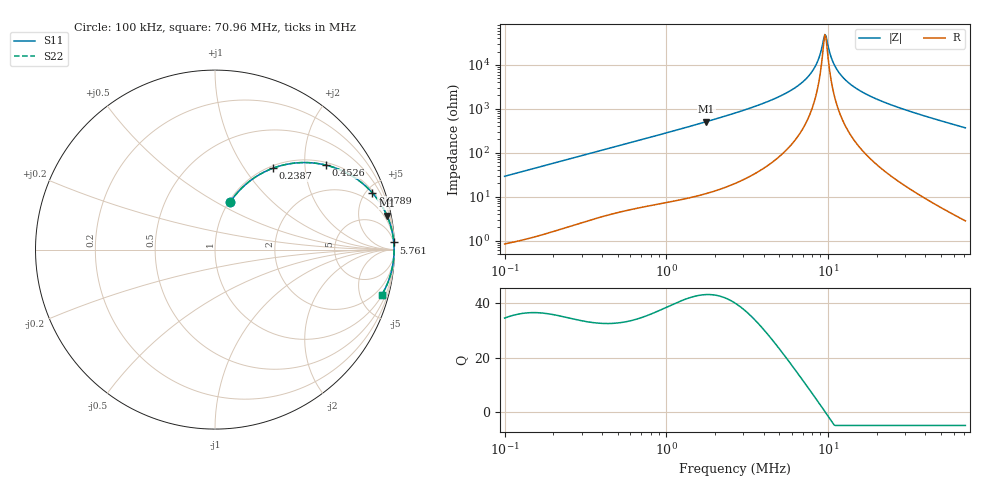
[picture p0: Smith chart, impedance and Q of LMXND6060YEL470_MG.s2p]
! LMXND6060YEL470_MG  S-PARAMETER MODEL  ( General Type )
! Model Generated by TAIYO YUDEN Corporation (http://www.ty-top.com)
! Version 1.0
! TAIYO YUDEN Control No. 191025NI43SB-FBB
! Copyright(c) 2019 TAIYO YUDEN CO.,LTD. All Rights Reserved.
! Product Description (link to TY-COMPAS)
! https://ds.yuden.co.jp/TYCOMPAS/or/detail?pn=LMXND6060YEL470MMG&u=M
! Products Name : Inductors
! Characteristics :
!  Inductance : 47 uH , SRF(min) : 5.0 MHz , DC Resistance(max) : 0.2743 Ohm
!  Rated Current : Saturation :1400 mA , Temp Rise : 1150 mA
!  Case Size : 6.0 x 6.0 / 0.236 x 0.236 [mm/inch] , Thickness : 4.5 / 0.177 [mm/inch]
!  (Conditions: Temperature = 25 degC , DC Bias Current/Voltage = 0A / 0V)
! External Node Assignments :
!  1  o---GGG---o  2
! GND o---------o GND
! Frequency Range : 0.1MHz  -  70.9631MHz  [ 402 STEP ]
# MHz S RI R 50
! Freq[MHz].  S11 Real  S11 Imag  S21 Real  S21 Imag  S12 Real  S12 Imag  S22 Real  S22 Imag
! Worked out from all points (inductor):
!   401 points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, 100 kHz to 70.96 MHz, reference 50 ohm
!   read as one part in series: L = 45.9 uH near 103.3 kHz
!   highest Q = 43.2 at 1.767 MHz (marker M1), where L = 45.5 uH
!   self-resonance near 9.582 MHz
!   S11 on the Smith chart (normalised r, x): 100 kHz: 1.02, +0.58; 238.7 kHz: 1.04, +1.37; 452.6 kHz: 1.08, +2.56; 978.9 kHz: 1.14, +5.50; 5.761 MHz: 4, +49; 70.96 MHz: 1.06, -7.33
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0.1  0.0837 0.2629  0.9163 -0.2629  0.9163 -0.2629  0.0837 0.2629
0.155756  0.1744 0.3661  0.8256 -0.3661  0.8256 -0.3661  0.1744 0.3661
0.23865  0.3237 0.4538  0.6763 -0.4538  0.6763 -0.4538  0.3237 0.4538
0.300295  0.4261 0.4798  0.5739 -0.4798  0.5739 -0.4798  0.4261 0.4798
0.452624  0.6184 0.4707  0.3816 -0.4707  0.3816 -0.4707  0.6184 0.4707
0.90177  0.8587 0.3352  0.1413 -0.3352  0.1413 -0.3352  0.8587 0.3352
0.97889  0.877 0.3156  0.123 -0.3156  0.123 -0.3156  0.877 0.3156
1.767367  0.9584 0.1885  0.0416 -0.1885  0.0416 -0.1885  0.9584 0.1885
2.70797  0.9821 0.1206  0.0179 -0.1206  0.0179 -0.1206  0.9821 0.1206
4.217825  0.9928 0.0688  0.00716 -0.0688  0.00716 -0.0688  0.9928 0.0688
5.761196  0.9962 0.0401  0.0038 -0.0401  0.0038 -0.0401  0.9962 0.0401
7.015257  0.9973 0.0241  0.00268 -0.0241  0.00268 -0.0241  0.9973 0.0241
7.999526  0.9978 0.014  0.00225 -0.014  0.00225 -0.014  0.9978 0.014
8.683647  0.9979 0.00773  0.00209 -0.00773  0.00209 -0.00773  0.9979 0.00773
9.426274  0.998 0.00156  0.00202 -0.00156  0.00202 -0.00156  0.998 0.00156
9.740813  0.998 -0.0009  0.00201 0.0009  0.00201 0.0009  0.998 -0.0009
10.40173  0.998 -0.00583  0.00203 0.00583  0.00203 0.00583  0.998 -0.00583
10.92668  0.9979 -0.00955  0.00208 0.00955  0.00208 0.00955  0.9979 -0.00955
12.66591  0.9976 -0.0209  0.00241 0.0209  0.00241 0.0209  0.9976 -0.0209
16.20131  0.9964 -0.0408  0.00363 0.0408  0.00363 0.0408  0.9964 -0.0408
24.02217  0.9919 -0.0781  0.0081 0.0781  0.0081 0.0781  0.9919 -0.0781
70.9631  0.9291 -0.2528  0.0709 0.2528  0.0709 0.2528  0.9291 -0.2528
